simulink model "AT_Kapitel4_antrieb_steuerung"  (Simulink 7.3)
settings: Solver=ode15s  StartTime=0.0  StopTime=60.0  RelTol=1e-3
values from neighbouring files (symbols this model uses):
  c_T = .2e-1    (= 0.02)    [set_data.m]
  d_T = 0    [set_data.m]
  k_A = .9    (= 0.9)    [set_data.m]
  L_A = 3/200    (= 0.015)    [set_data.m]
  R_A = 20    [set_data.m]
  theta_G = .3500000000e-2    (= 0.0035)    [set_data.m]
  theta_L = .6300000000e-2    (= 0.0063)    [set_data.m]
libraries: cstblocks x1

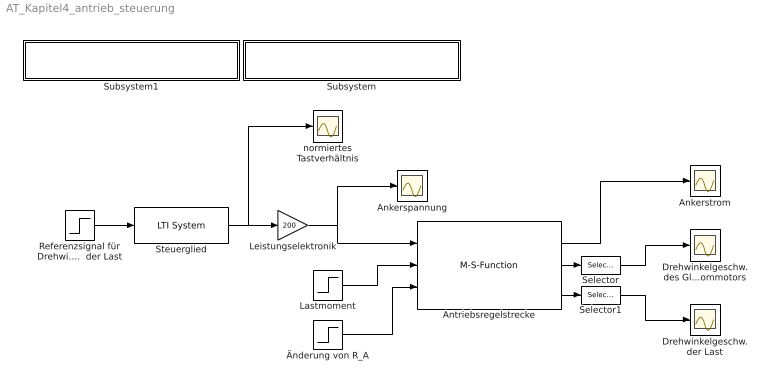
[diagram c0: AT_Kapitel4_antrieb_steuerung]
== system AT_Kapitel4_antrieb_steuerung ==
  Ankerspannung : Scope
  Ankerstrom : Scope
  Antriebsregelstrecke : M-S-Function  FunctionName=Antrieb_S_m  Parameters=RAp,LAp,kAp,thetaGp,thetaLp,cTp,dTp  mask{RAp=R_A, LAp=L_A, kAp=k_A, thetaGp=theta_G, thetaLp=theta_L, cTp=c_T, dTp=d_T}
      mask prompts: RAp "Ankerwiderstand"; LAp "Ankerinduktivität"; kAp "Ankerkreiskonstante"; thetaGp "Trägheitsmoment GSM"; thetaLp "Trägheitsmoment Last"; cTp "Federsteifigkeit"; dTp "Dämpfungskonstante"
  Drehwinkelgeschw. der Last : Scope
  Drehwinkelgeschw. des Gleichstrommotors : Scope
  Lastmoment : Step  Time=20  SampleTime=0
  Leistungselektronik : Gain  Gain=200  ParameterDataType=sfix(16)  ParameterScaling=2^0  OutDataType=sfix(16)  OutScaling=2^0
  Referenzsignal für Drehwinkelgeschw.  der Last : Step  Time=10  Before=100  After=-100  SampleTime=0
  Selector : Selector  InputPortWidth=2  IndexOptions=Index vector (dialog)  Indices=[2]  OutputSizes=1
  Selector1 : Selector  InputPortWidth=2  IndexOptions=Index vector (dialog)  Indices=[2]  OutputSizes=1
  Steuerglied : cstblocks/LTI System  SystemSampleTime=-1  sys=R1  IC=[]
  Subsystem : Subsystem  Description=test
  Subsystem1 : Subsystem  Description=test
  normiertes Tastverhältnis : Scope
  Änderung von R_A : Step  Time=40  Before=1  After=1.4  SampleTime=0
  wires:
  Referenzsignal für Drehwinkelgeschw.  der Last/1 -> Steuerglied/1
  Lastmoment/1 -> Antriebsregelstrecke/2
  Steuerglied/1 -> Leistungselektronik/1, normiertes Tastverhältnis/1
  Leistungselektronik/1 -> Ankerspannung/1, Antriebsregelstrecke/1
  Änderung von R_A/1 -> Antriebsregelstrecke/3
  Antriebsregelstrecke/1 -> Ankerstrom/1
  Antriebsregelstrecke/2 -> Selector/1
  Selector/1 -> Drehwinkelgeschw. des Gleichstrommotors/1
  Antriebsregelstrecke/3 -> Selector1/1
  Selector1/1 -> Drehwinkelgeschw. der Last/1

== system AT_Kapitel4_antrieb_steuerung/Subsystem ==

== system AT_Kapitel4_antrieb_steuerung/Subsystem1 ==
